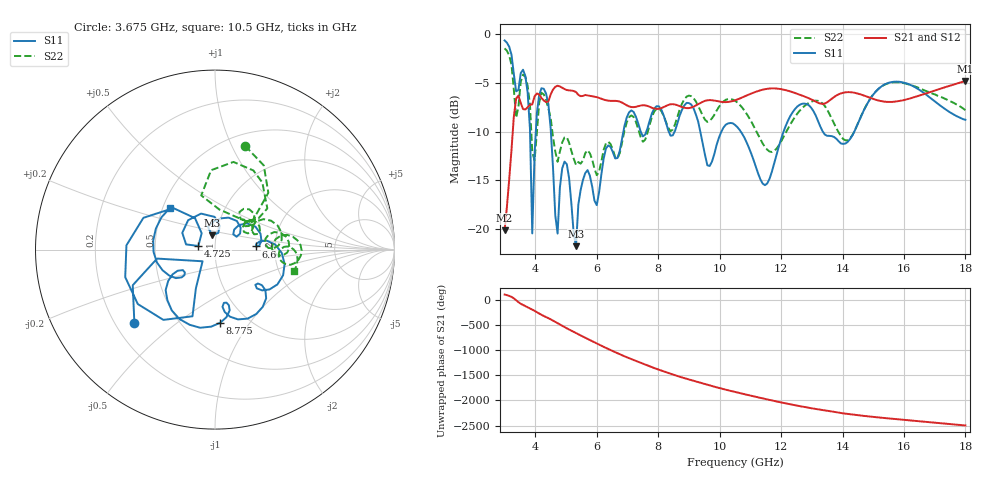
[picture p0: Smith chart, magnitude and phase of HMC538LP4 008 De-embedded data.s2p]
! Chelmsford, MA 01824
! http://www.hittite.com
! Tel: 978-250-3343
! Fax: 978-250-3373
! Device  :  HMC538LP4
! Description:  600 Analog Phase Shifter
! Frequency  :  6.0 GHz - 15.0 GHz
! Package  :  LP4  - 4x4 mm Quad Flatpack No-Lead (QFN) Plastic Package: 24 pin
! Ports  :  2 RF, 1 DC
!  Pin  3  = Rfin  = Port 1
!  Pin  16  = Rfout = Port 2
!  pin  21  = vCTL
! Voltages:  VCTL  = 0 to 5.0 Volts
! Currents :  Vb(V)  Vd(V)  Ib(mA)  Id(mA)
!  0.00  0.80  0.000000	0.483525
! Data:  The device was measured on evaluation board 111296-1.
!  Data was collected using a calibrated network analyzer.
!  The evaluation circuit board was modeled and simulated.This was use
!  to removed the evaluation board circuit from the measured data.
!  The reference plane is the center of the package pin.
! Misc:  Lot #
!Date Measured:  03 - 11 -2009
! Date:  03 - 17 -2009
! Note:
!  Hittite Microwave supplies this data as a sample of measured data at the
!  package pin for this package product.  Your particular data for this product
!  may vary.
!  Data was taken at 25 degrees C.
!  Hittite Microwave reserves the right to change this data at anytime.
# MHz S MA R 50
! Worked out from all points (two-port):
!   201 points, 3 GHz to 18 GHz, reference 50 ohm
!   highest |S21| = -4.83 dB at 18 GHz (marker M1); lowest = -20.1 dB at 3 GHz (marker M2)
!   |S21| within 3 dB of the highest: 3.327 GHz to end of sweep
!   lowest |S11| = -21.7 dB at 5.325 GHz (marker M3), VSWR 1.18, Z = 47.7 + j7.71 ohm
!   |S11| at or under -10 dB: 4.506 GHz to 6.867 GHz (2.362 GHz wide, 41.5 % of centre); 10.69 GHz to 12.08 GHz (1.396 GHz wide, 12.3 % of centre); 13.36 GHz to 14.38 GHz (1.027 GHz wide, 7.41 % of centre)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
!   |S22| runs from -14.5 to -1.5 dB; largest |S21 - S12| = 0.0017
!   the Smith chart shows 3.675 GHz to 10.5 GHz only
!   S11 on the Smith chart (normalised r, x): 3.675 GHz: 0.28, -0.36; 4.725 GHz: 0.83, +0.03; 6.6 GHz: 1.59, +0.06; 8.775 GHz: 0.75, -0.74; 10.5 GHz: 0.55, +0.29
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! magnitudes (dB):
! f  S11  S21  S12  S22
! 3 GHz  -0.7  -20.1  -20.1  -1.5
! 3.375 GHz  -5.9  -6.6  -6.6  -8.6
! 3.675 GHz  -4.3  -7.7  -7.7  -4.4
! 3.825 GHz  -9.7  -7.3  -7.3  -7.2
! 3.9 GHz  -20.4  -7.2  -7.2  -12.1
! 4.05 GHz  -8.1  -6.1  -6.1  -10.1
! 4.2 GHz  -5.6  -6.6  -6.6  -6.0
! 4.425 GHz  -7.2  -6.9  -6.9  -7.7
! 4.725 GHz  -20.4  -5.3  -5.3  -13.1
! 4.95 GHz  -13.1  -5.7  -5.7  -10.6
! 5.325 GHz  -21.7  -6.0  -6.0  -13.4
! 5.55 GHz  -15.0  -6.4  -6.4  -13.0
! 6.6 GHz  -12.8  -6.9  -6.9  -12.6
! 8.025 GHz  -7.4  -7.7  -7.7  -7.7
! 8.775 GHz  -7.8  -7.5  -7.5  -7.1
! 9.675 GHz  -13.5  -6.8  -6.8  -8.9
! 10.5 GHz  -9.3  -6.8  -6.8  -6.8
! 11.47 GHz  -15.5  -5.7  -5.7  -11.6
! 13.05 GHz  -7.9  -6.8  -6.8  -6.9
! 14.18 GHz  -11.0  -6.0  -6.0  -10.9
! 15.53 GHz  -5.0  -7.0  -7.0  -5.0
! 18 GHz  -8.8  -4.8  -4.8  -7.8
